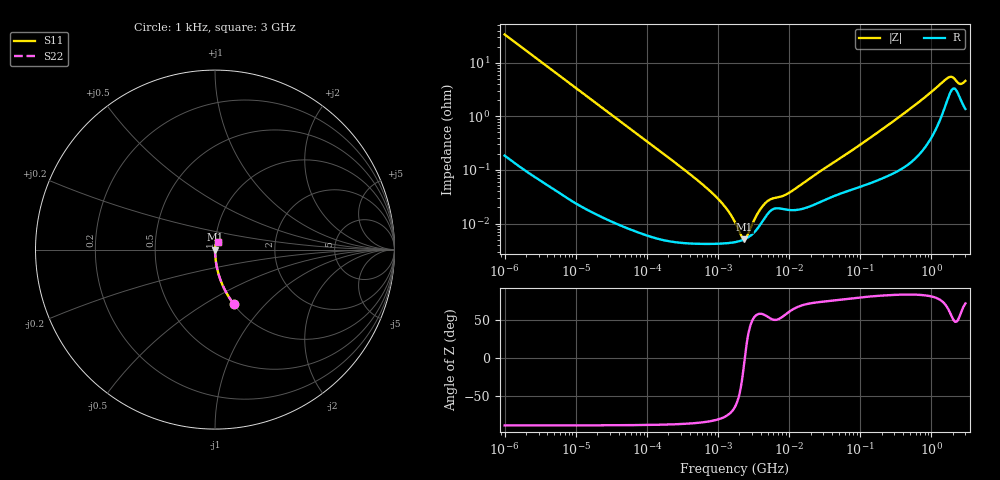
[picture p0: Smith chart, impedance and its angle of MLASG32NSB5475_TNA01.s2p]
! MLASG32NSB5475_TNA01  S-PARAMETER MODEL  ( Standard Model )
! Model Generated by TAIYO YUDEN Corporation (http://www.ty-top.com)
! Version 1.0
! TAIYO YUDEN Control No. 220601
! Copyright(c) 2009 TAIYO YUDEN CO.,LTD. All Rights Reserved.
! Product Description (link to TY-COMPAS)
! https://ds.yuden.co.jp/TYCOMPAS/or/detail?pn=MLASG32NSB5475KTNA01&u=M
! Products Name : Multilayer Ceramic Capacitors
! Characteristics :
!  Capacitance : 4.7 [uF] , Rated Voltage : 35 [V] , TCC : X5R
!  Case Size : 3.2 x 2.5 / 0.126 x 0.098 [mm/inch] , Thickness : 1.9 / 0.075 [mm/inch]
!  (Conditions: Temperature = 25 [degC] , DC Bias Voltage = 0 [V])
! External Node Assignments :
!  1  o---| |---o  2
! GND o---------o GND
! Frequency Range : 1kHz  -  3GHz  [ 401 STEP ]
# MHZ S RI R 50
! Freq[MHz].  S11 Real  S11 Imag  S21 Real  S21 Imag  S12 Real  S12 Imag  S22 Real  S22 Imag
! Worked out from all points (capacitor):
!   401 points, 1 kHz to 3 GHz, reference 50 ohm
!   read as one part in series: C = 4.71 uF near 1.077 kHz
!   lowest |Z| = 5.08 mohm at 2.334 MHz (marker M1)
!   series resonance near 2.379 MHz, so ESL is about 950 pH
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0.001  0.1036 -0.302  0.8964 0.302  0.8964 0.302  0.1036 -0.302
0.001685  0.0397 -0.1924  0.9603 0.1924  0.9603 0.1924  0.0397 -0.1924
0.00306  0.0127 -0.1092  0.9873 0.1092  0.9873 0.1092  0.0127 -0.1092
0.01216  0.000987 -0.028  0.999 0.028  0.999 0.028  0.000987 -0.028
0.147855  5.65e-05 -0.00232  0.9999 0.00232  0.9999 0.00232  5.65e-05 -0.00232
0.43594  4.27e-05 -0.000765  1 0.000765  1 0.000765  4.27e-05 -0.000765
0.821683  4.18e-05 -0.000372  1 0.000372  1 0.000372  4.18e-05 -0.000372
1.238299  4.26e-05 -0.000206  1 0.000206  1 0.000206  4.26e-05 -0.000206
1.732051  4.49e-05 -9.58e-05  1 9.58e-05  1 9.58e-05  4.49e-05 -9.58e-05
1.937042  4.64e-05 -6.18e-05  1 6.18e-05  1 6.18e-05  4.64e-05 -6.18e-05
2.334012  5.04e-05 -5.75e-06  0.9999 5.75e-06  0.9999 5.75e-06  5.04e-05 -5.75e-06
3.03007  6.31e-05 7.49e-05  0.9999 -7.49e-05  0.9999 -7.49e-05  6.31e-05 7.49e-05
4.083148  0.000103 0.00017  0.9999 -0.00017  0.9999 -0.00017  0.000103 0.00017
5.106836  0.000157 0.000218  0.9998 -0.000218  0.9998 -0.000218  0.000157 0.000218
9.273352  0.000181 0.000304  0.9998 -0.000304  0.9998 -0.000304  0.000181 0.000304
21.06097  0.000217 0.000714  0.9998 -0.000714  0.9998 -0.000714  0.000217 0.000714
256.0921  0.000843 0.00711  0.9992 -0.00711  0.9992 -0.00711  0.000843 0.00711
700.8126  0.00243 0.0193  0.9976 -0.0193  0.9976 -0.0193  0.00243 0.0193
1652.1  0.0209 0.0454  0.9791 -0.0454  0.9791 -0.0454  0.0209 0.0454
1917.819  0.0317 0.0425  0.9683 -0.0425  0.9683 -0.0425  0.0317 0.0425
2489.759  0.0233 0.0319  0.9767 -0.0319  0.9767 -0.0319  0.0233 0.0319
3000  0.0154 0.0426  0.9846 -0.0426  0.9846 -0.0426  0.0154 0.0426
